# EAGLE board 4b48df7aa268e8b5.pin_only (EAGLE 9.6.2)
REV: C

Size 53.34 x 68.58 mm. Coordinates in mm from the lower left corner, seen from the top.
Outline: 53.34,4.06 51.82,2.54 40.39,2.54 37.85,0 5.08,0 2.54,2.54 1,2.54 arc-90 0,3.54 0,43.81 0.89,44.7 0.89,49.66 0,50.55 0,67.58 arc-90 1,68.58 52.34,68.58 arc-90 53.34,67.58 53.34,4.06
Copper layers (1*16): Top 0.035mm / dielectric 1.5mm / Bottom 0.035mm
Design rules "adafruit *": minimum track width 8mil, minimum drill 15.5mil, track to track 8mil, track to pad 8mil, pad to pad 8mil, via to via 8mil, smd to smd 8mil, copper to edge 10mil, drill to drill 8mil, minimum pad ring 10mil, minimum via ring 8mil, stop-mask expansion 2mil, vias tented up to drill 20mil, thermal gap 10mil
Net classes: 2 lowpower: width 0.305 mm, drill 0.483 mm; 3 Power: width 0.305 mm, drill 0.483 mm
Holes 3.2 mm at 35.56,2.54 7.62,2.54 50.8,53.34 2.54,54.61

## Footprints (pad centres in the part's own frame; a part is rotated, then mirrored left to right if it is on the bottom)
1X06_OVALWAVE = drill 0.8 pad 1.5 long: 1 -6.35,0; 2 -3.81,0; 3 -1.27,0; 4 1.27,0; 5 3.81,0; 6 6.35,0
0805-NO = smd 1.24 x 1.5: 1 -0.95,0; 2 0.95,0
0603-NO = smd 1.075 x 1: 1 -0.85,0; 2 0.85,0
CHIPLED_0603_NOOUTLINE = smd 0.8 x 0.8: A 0,-0.75; C 0,0.75
JST_SH4 = smd 0.6 x 1.55: 1 -1.5,2.514; 2 -0.5,2.514; 3 0.5,2.514; 4 1.5,2.514 | smd 1.2 x 1.8: MT1 -2.8,-1.386; MT2 2.8,-1.386
SOD-123 = smd 1.4 x 1.4: A 1.85,0; C -1.85,0
1206 = smd 1.6 x 1.8: 1 -1.4,0; 2 1.4,0
FIDUCIAL_1MM = smd 1 x 1: 1 0,0
WDFN8_3X4_0.65 = smd 0.7 x 0.35: 1 -1.8,0.975; 2 -1.8,0.325; 3 -1.8,-0.325; 4 -1.8,-0.975; 5 1.8,-0.975; 6 1.8,-0.325; 7 1.8,0.325; 8 1.8,0.975 | smd 2.3 x 1.96: P$9 0,0
2X03_ROUND_70MIL = drill 0.9 pad 1.778: 1 -2.54,-1.27; 2 -2.54,1.27; 3 0,-1.27; 4 0,1.27; 5 2.54,-1.27; 6 2.54,1.27
1X10_OVALWAVE = drill 0.8 pad 1.5 long: 1 -11.43,0; 2 -8.89,0; 3 -6.35,0; 4 -3.81,0; 5 -1.27,0; 6 1.27,0; 7 3.81,0; 8 6.35,0; 9 8.89,0; 10 11.43,0
1X08_OVALWAVE = drill 0.8 pad 1.5 long: 1 -8.89,0; 2 -6.35,0; 3 -3.81,0; 4 -1.27,0; 5 1.27,0; 6 3.81,0; 7 6.35,0; 8 8.89,0
1X02_ROUND = drill 1 pad 1.778: 1 -1.27,0; 2 1.27,0
LED3535 = smd 1 x 0.85: 1 -1.75,0.875; 2 -1.75,-0.875; 3 1.75,-0.875; 4 1.75,0.875
PANASONIC_D = smd 3.556 x 1.4: + 2.654,0; - -2.654,0
SOT23-R = smd 0.635 x 1.016: 1 -0.95,-1; 2 0.95,-1; 3 0,1
RESPACK_4X0603 = smd 0.45 x 0.9: 1 -1.3,-0.85; 2 -0.4,-0.85; 3 0.4,-0.85; 4 1.3,-0.85; 5 1.3,0.85; 6 0.4,0.85; 7 -0.4,0.85; 8 -1.3,0.85
SOLDERJUMPER_CLOSEDWIRE = smd 1.168 x 1.6: 1 -0.762,0; 2 0.762,0 | smd 0.635 x 0.203: WIRE 0,0
SPST_TACTILE_RA = smd 0.9 x 1.27: 1 -2.1,0.9; 2 2.1,0.9 | smd 1.45 x 0.8: MT1 -3.375,-1; MT2 3.375,-1 | hole 1: -1.15,-0.3; 1.15,-0.3
SPDT_SMT_SSSS811101 = smd 0.7 x 1.5: A -2.25,1.75; B 0.75,1.75; C 2.25,1.75 | smd 1 x 0.8: SUP1 -3.65,1.1; SUP2 -3.65,-1.1; SUP3 3.65,1.1; SUP4 3.65,-1.1 | hole 0.9: -1.5,0; 1.5,0
TESTPOINT_ROUND_1.5MM_NO = smd 1.5 x 1.5: P$1 0,0
SOT223-R = smd 1.3 x 1.3: 1 -2.3,-3.05; 2 0,-3.05; 3 2.3,-3.05 | smd 3.6 x 1.3: 4 0,3.05
SOT23-5 = smd 0.55 x 1.2: 1 -0.95,-1.3; 2 0,-1.3; 3 0.95,-1.3; 4 0.95,1.3; 5 -0.95,1.3
MODULE_ESP32-S2-WROVER = smd 1.5 x 0.9: 1 -8.75,8; 2 -8.75,6.5; 3 -8.75,5; 4 -8.75,3.5; 5 -8.75,2; 6 -8.75,0.5; 7 -8.75,-1; 8 -8.75,-2.5; 9 -8.75,-4; 10 -8.75,-5.5; 11 -8.75,-7; 12 -8.75,-8.5; 13 -8.75,-10; 14 -8.75,-11.5; 15 -8.75,-13; 16 -8.75,-14.5; 27 8.75,-14.5; 28 8.75,-13; 29 8.75,-11.5; 30 8.75,-10; 31 8.75,-8.5; 32 8.75,-7; 33 8.75,-5.5; 34 8.75,-4; 35 8.75,-2.5; 36 8.75,-1; 37 8.75,0.5; 38 8.75,2; 39 8.75,3.5; 40 8.75,5; 41 8.75,6.5; 42 8.75,8 | smd 0.9 x 1.5: 17 -6.75,-15.25; 18 -5.25,-15.25; 19 -3.75,-15.25; 20 -2.25,-15.25; 21 -0.75,-15.25; 22 0.75,-15.25; 23 2.25,-15.25; 24 3.75,-15.25; 25 5.25,-15.25; 26 6.75,-15.25 | smd 1.1 x 1.1: 43_1 -2.69,1.45; 43_2 -1.19,1.45; 43_3 0.31,1.45; 43_4 -2.69,-0.05; 43_5 -1.19,-0.05; 43_6 0.31,-0.05; 43_7 -2.69,-1.55; 43_8 -1.19,-1.55; 43_9 0.31,-1.55 | drill 0.4: 43_10 -1.94,1.45; 43_11 -0.44,1.45; 43_12 -2.69,0.7; 43_13 -1.19,0.7; 43_14 0.31,0.7; 43_15 -1.94,-0.05; 43_16 -0.44,-0.05; 43_17 -2.69,-0.8; 43_18 -1.19,-0.8; 43_19 0.31,-0.8; 43_20 -1.94,-1.55; 43_21 -0.44,-1.55
JSTPH2_BATT = smd 1 x 4.6: 1 -1,-3.7; 2 1,-3.7 | smd 1.6 x 3.4: NC1 -3.4,1.5; NC2 3.4,1.5
2X05_1.27MM_BOX_POSTS = smd 0.76 x 2.6: 1 -2.54,-2.15; 2 -2.54,2.15; 3 -1.27,-2.15; 4 -1.27,2.15; 5 0,-2.15; 6 0,2.15; 7 1.27,-2.15; 8 1.27,2.15; 9 2.54,-2.15; 10 2.54,2.15 | hole 1: -1.905,0; 1.905,0
USB_C_CUSB31-CFM2AX-01-X = smd 0.575 x 1.15: A1B12 -3.2,3.545; A4B9 -2.4,3.545; B1A12 3.2,3.545; B4A9 2.4,3.545 | smd 0.275 x 1.15: A5 -1.25,3.545; A6 -0.25,3.545; A7 0.25,3.545; A8 1.25,3.545; B5 1.75,3.545; B6 0.75,3.545; B7 -0.75,3.545; B8 -1.75,3.545 | drill 0.6 pad 1 long: M1 -4.32,2.97; M2 4.32,2.97; M3 -4.32,-1.21; M4 4.32,-1.21 | hole 0.65: 2.89,2.47; -2.89,2.47
DCJACK_2MM_PTH = drill 0.9 pad 2.7 long: GND 7.35,0; GNDBREAK 10.75,-4.8; PWR 13.6,0

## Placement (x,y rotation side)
AD  20609  [1X06_OVALWAVE]  2.54,11.43 270 top
C1  10uF  [0805-NO]  38.29,55.94 180 top
C2  0.1uF  [0603-NO]  44.7,42.35 270 top
C3  10uF  [0805-NO]  19.3,20.38 90 top
C4  10µF  [0805-NO]  28.45,21.46 90 top
C5  0.1uF  [0603-NO]  30.23,17.91 270 top
C6  1uF  [0603-NO]  37.46,43.24 270 top
C7  10µF  [0805-NO]  10.03,55.63 180 top
C8  10µF  [0805-NO]  16.13,11.11 0 top
C10  10µF  [0805-NO]  9.53,53.72 180 top
C11  10µF  [0805-NO]  18.92,17.59 180 top
C12  0.1uF  [0603-NO]  19.18,23.81 90 top
C13  10µF  [0805-NO]  28.51,17.91 270 top
C14  1uF  [0603-NO]  43.56,58.48 270 top
C15  0.1uF  [0603-NO]  43.56,55.37 90 top
C17  10µF  [0805-NO]  8.76,51.82 180 top
C18  10µF  [0805-NO]  7.75,49.91 180 top
CHG1  ORANGE  [CHIPLED_0603_NOOUTLINE]  40.07,8.23 0 top
CONN1  STEMMA_I2C_QT  [JST_SH4]  50.8,60.07 90 top
D1  MBR540  [SOD-123]  6.22,53.78 90 top
D4  MBR540  [SOD-123]  21.59,19.49 90 top
F2  500mA  [1206]  41.59,57.59 270 top
FD1  FIDUCIAL_1MM  [FIDUCIAL_1MM]  52.07,65.28 270 top
FD2  FIDUCIAL_1MM  [FIDUCIAL_1MM]  4.68,2.55 270 top
FD3  FIDUCIAL_1MM  [FIDUCIAL_1MM]  1.89,66.63 270 top
IC2  LC709203F  [WDFN8_3X4_0.65]  21.72,9.65 0 top
ICSP  3x2 M  [2X03_ROUND_70MIL]  27.94,3.94 180 top
IOH  20611  [1X10_OVALWAVE]  50.8,38.35 270 top
IOL  20610  [1X08_OVALWAVE]  50.8,13.97 270 top
JP2  UART  [1X02_ROUND]  33.53,54.23 90 top
L  RED  [CHIPLED_0603_NOOUTLINE]  42.47,8.27 180 top
LED1  WS2812B3535  [LED3535]  41.91,42.54 270 top
ON  GREEN  [CHIPLED_0603_NOOUTLINE]  44.42,8.22 180 top
PC1  47uF/25V  [PANASONIC_D]  10.35,29.46 90 top
PC2  47uF+/6.3V+  [PANASONIC_D]  13.72,15.43 180 top
POWER  20610  [1X08_OVALWAVE]  2.54,31.75 270 top
Q1  DMG3415U-7  [SOT23-R]  20.07,14.92 90 top
Q2  DMG3415U-7  [SOT23-R]  24.83,22.1 270 top
R1  10K  [RESPACK_4X0603]  45.85,54.48 90 top
R2  10K  [0603-NO]  40.26,12.81 90 top
R3  5.1K  [0603-NO]  35.88,56.9 90 top
R4  2.2K  [0603-NO]  11.24,6.86 270 top
R6  10K  [0603-NO]  43.56,16.12 90 top
R8  5.1K  [0603-NO]  38.16,58.23 0 top
R9  10K  [0603-NO]  42.04,14.08 90 top
R12  100K  [0603-NO]  23.69,15.49 180 top
R14  100k  [0603-NO]  23.69,13.21 180 top
R15  100K  [0603-NO]  20.76,23.81 270 top
R16  100K  [0603-NO]  22.35,23.81 270 top
R17  1Meg  [0603-NO]  39.05,43.24 90 top
SJ1  [SOLDERJUMPER_CLOSEDWIRE]  38.99,43.94 0 bottom
SW1  RA_TACT  [SPST_TACTILE_RA]  42.47,4.38 0 top
SW3  RA_TACT  [SPST_TACTILE_RA]  47.37,66.8 180 top
SW4  SPDT R/A  [SPDT_SMT_SSSS811101]  2.54,47.12 270 top
TP1  [TESTPOINT_ROUND_1.5MM_NO]  12.06,50.67 0 bottom
U1  NCP1117ST50T3G  [SOT223-R]  14.22,22.42 90 top
U2  MCP73831T-2ACI/OT  [SOT23-5]  12.32,10.22 90 top
U3  ESP32-S2-WROVER  [MODULE_ESP32-S2-WROVER]  22.67,52.96 0 top
U4  AP2112(3.3V)  [SOT23-5]  25.27,17.97 270 top
U$15  [PCBFEAT-REV-040]  29.34,14.29 270 top
U$52  [ESP32S2_TOP]  0,68.58 270 top
U$53  [ESP32S2_BOT]  0,0 90 bottom
X1  JSTPH  [JSTPH2_BATT]  16.13,3.49 180 top
X2  4u20317  [2X05_1.27MM_BOX_POSTS]  39.5,49.66 0 top
X4  USB C  [USB_C_CUSB31-CFM2AX-01-X]  38.1,64.77 180 top
X5  2.1mm  [DCJACK_2MM_PTH]  8.13,71.88 270 top

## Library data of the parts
AD C1-C8 C10-C15 C17 C18 CHG1 CONN1 D1 D4 F2 IC2 ICSP IOH IOL JP2 L LED1 ON PC1 PC2 POWER Q1 Q2 R1-R4 R6 R8 R9 R12 R14-R17 SJ1 SW1 SW3 SW4 TP1 U1 U2 U4 U$15 X1 X2 X4 X5 = microbuilder
FD1-FD3 = microbuilder; BOM: EXCLUDE
U3 = adafruit_wireless; AVAILABILITY: Warning; DESCRIPTION: WiFi 802.11b/g/n Transceiver Module 2.4GHz Antenna Not Included Surface Mount; DIGIKEY-PURCHASE-URL: https://snapeda.com/shop?store=DigiKey&id=4614060; MF: Espressif Systems; MP: ESP32-S2-WROVER; PACKAGE: VFQFN-56 Espressif Systems; PRICE: None
U$52 U$53 = metro_silks

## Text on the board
214bmp: D:/SmartProjects/Snc/a4_bn_logo2.bmp

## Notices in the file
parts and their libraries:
microbuilder: This work is placed in the public domain, and may be freely used for commercial and non-commercial work with the following conditions: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
